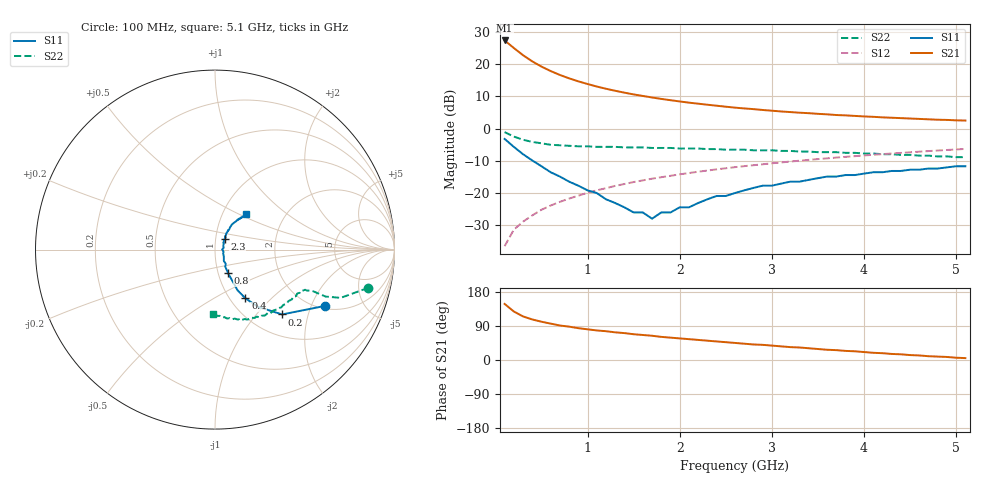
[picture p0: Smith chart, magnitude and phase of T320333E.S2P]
!AT-32033
!S PARAMETERS at Vce=2.7V  Ic=10mA.  LAST UPDATED 01-05-95
# ghz s ma r 50
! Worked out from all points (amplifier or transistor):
!   51 points, 100 MHz to 5.1 GHz, reference 50 ohm
!   highest |S21| = 27.3 dB at 100 MHz (marker M1)
!   |S21| within 3 dB of that: start of sweep to 229.5 MHz
!   unconditionally stable (mu >= 1): 1.022 GHz to 2.192 GHz; 2.213 GHz to 2.366 GHz; 2.443 GHz to 2.542 GHz
!   at 900 MHz: K = 1.00, MSG = 17.7 dB, |S12| = -20.8 dB
!   at 2.6 GHz: K = 1.00, MSG = 9.2 dB, |S12| = -12.0 dB
!   at 5.1 GHz: K = 0.93, MSG = 4.4 dB, |S12| = -6.3 dB
!   S11 on the Smith chart (normalised r, x): 100 MHz: 2.13, -2.54; 200 MHz: 1.40, -1.38; 400 MHz: 1.18, -0.71; 800 MHz: 1.11, -0.30; 2.3 GHz: 1.10, +0.13; 5.1 GHz: 1.28, +0.54
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0.1  0.69 -27.0  23.21 148.0  0.015 77.0  0.88 -14.0
0.2  0.52 -44.0  17.73 128.0  0.027 73.0  0.75 -21.0
0.3  0.4 -53.0  13.7 115.0  0.036 71.0  0.67 -23.0
0.4  0.32 -58.0  11 107.0  0.045 72.0  0.62 -23.0
0.5  0.26 -61.0  9.13 101.0  0.055 72.0  0.59 -23.0
0.6  0.21 -61.0  7.78 96.0  0.064 72.0  0.56 -24.0
0.7  0.18 -61.0  6.77 91.0  0.073 72.0  0.55 -24.0
0.8  0.15 -61.0  6 88.0  0.082 72.0  0.54 -25.0
0.9  0.13 -60.0  5.39 84.0  0.091 71.0  0.53 -26.0
1  0.11 -59.0  4.9 81.0  0.101 71.0  0.53 -27.0
1.1  0.1 -53.0  4.48 78.0  0.11 70.0  0.52 -28.0
1.3  0.07 -45.0  3.85 73.0  0.129 69.0  0.52 -30.0
1.5  0.05 -25.0  3.38 68.0  0.148 67.0  0.51 -32.0
1.6  0.05 -16.0  3.2 66.0  0.157 67.0  0.51 -33.0
1.7  0.04 2.0  3.03 64.0  0.167 66.0  0.5 -35.0
1.8  0.05 13.0  2.88 61.0  0.176 65.0  0.5 -36.0
2.1  0.06 39.0  2.52 55.0  0.204 62.0  0.49 -40.0
2.3  0.08 48.0  2.34 51.0  0.223 60.0  0.48 -43.0
2.6  0.1 53.0  2.11 45.0  0.252 57.0  0.47 -47.0
3.5  0.17 56.0  1.69 29.0  0.336 47.0  0.43 -62.0
4.3  0.22 52.0  1.47 16.0  0.41 38.0  0.4 -76.0
5.1  0.26 49.0  1.33 5.0  0.483 29.0  0.36 -92.0
